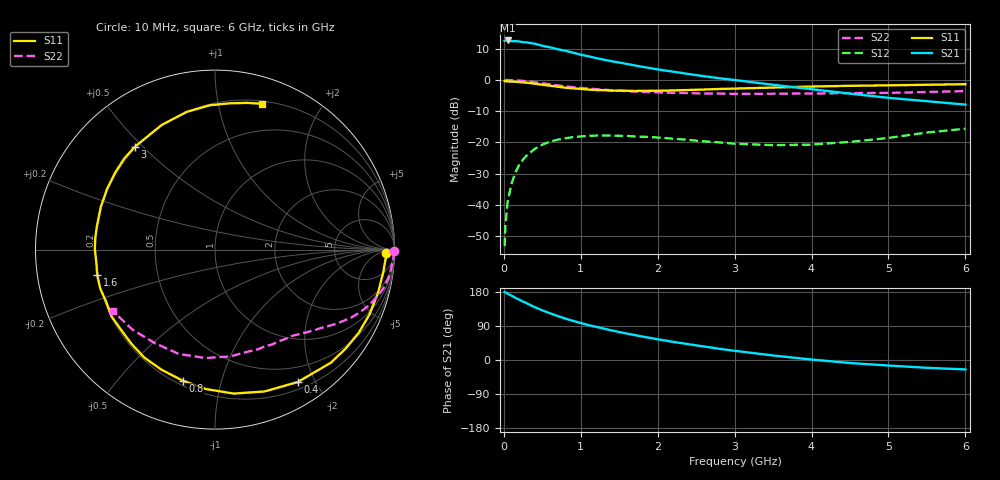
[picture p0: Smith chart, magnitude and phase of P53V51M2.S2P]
! SIEMENS Small Signal Semiconductors
! BFP183
! Si NPN RF Bipolar Junction Transistor in SOT143
! VCE = 3.5 V  IC = 1.2 mA
! Common Emitter S-Parameters:  March  1996
# GHz  S  MA  R  50
!  f  S11  S21  S12  S22
! GHz  MAG  ANG  MAG  ANG  MAG  ANG  MAG  ANG
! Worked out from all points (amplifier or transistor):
!   36 points, 10 MHz to 6 GHz, reference 50 ohm
!   highest |S21| = 12.6 dB at 50 MHz (marker M1)
!   |S21| within 3 dB of that: start of sweep to 738.5 MHz
!   unconditionally stable (mu >= 1): 2.421 GHz to end of sweep
!   at 250 MHz: K = 0.09, MSG = 18.7 dB, |S12| = -25.4 dB
!   at 1.4 GHz: K = 0.56, MSG = 11.9 dB, |S12| = -17.8 dB
!   at 6 GHz: K = 1.02, MAG = 3.0 dB, |S12| = -15.6 dB
!   S11 on the Smith chart (normalised r, x): 10 MHz: 35, -18; 400 MHz: 0.29, -1.77; 800 MHz: 0.23, -0.76; 1.6 GHz: 0.20, -0.10; 3 GHz: 0.20, +0.47; 6 GHz: 0.22, +1.35
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0.01  0.9557 -1.3  4.206 179.3  0.0022 91.1  0.9999 -0.5
0.02  0.9522 -3.0  4.256 178.5  0.0046 86.9  0.9947 -1.0
0.05  0.946 -7.7  4.274 174.8  0.0115 86.1  0.9952 -2.6
0.1  0.9397 -14.9  4.154 169.6  0.0219 80.6  0.9882 -5.3
0.15  0.9332 -22.9  4.176 164.2  0.0332 76.5  0.9841 -8.0
0.2  0.9255 -29.9  4.12 159.0  0.0437 72.3  0.9741 -10.5
0.3  0.9022 -44.3  3.977 149.5  0.0625 64.2  0.9473 -15.1
0.4  0.8702 -58.0  3.793 139.6  0.0787 56.5  0.9165 -19.5
0.5  0.8374 -70.7  3.514 131.0  0.092 49.3  0.8823 -23.1
0.6  0.8092 -82.5  3.319 123.3  0.1035 42.9  0.8507 -26.3
0.8  0.7516 -103.9  2.92 109.2  0.1168 32.7  0.7911 -31.5
1  0.7191 -123.2  2.526 97.6  0.1246 24.0  0.744 -35.6
1.1  0.7014 -131.7  2.389 92.0  0.1274 20.7  0.7259 -37.4
1.3  0.6862 -147.2  2.105 82.7  0.1295 14.1  0.6973 -40.8
1.6  0.6712 -167.7  1.801 69.7  0.1273 7.3  0.663 -45.4
1.8  0.6693 180.0  1.62 61.8  0.1238 4.1  0.6433 -48.6
2.2  0.6793 159.6  1.354 47.9  0.1149 -0.7  0.6218 -55.3
3  0.7264 127.8  0.997 24.3  0.0956 -0.3  0.5983 -71.0
3.5  0.7554 113.1  0.836 11.9  0.0905 6.3  0.6013 -82.0
4.5  0.8051 91.9  0.604 -8.0  0.1021 21.3  0.6154 -109.2
5.5  0.8366 77.7  0.457 -20.6  0.1443 26.3  0.6407 -136.0
6  0.8542 72.0  0.403 -24.9  0.166 23.3  0.663 -148.7
